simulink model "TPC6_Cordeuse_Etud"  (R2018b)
settings: Solver=ode23t  StartTime=0.0  StopTime=5  RelTol=1e-3  EnableMultiTasking=on
model workspace (MAT data in the model file):
  J = 0
  K1 = 0.561
  Kcan = 51
  Kcorde = 5052
  Ke = 0.024
  Kh = 0.0705882352941
  Ki = 0
  Kinc = 0
  Kp = 2
  Kpc = 0
  Kpot = 0.333333333333
  Kr = 0
  Kress = 0.033
  L = 0.02
  R = 0.7
  f = 0
libraries: simulink x1

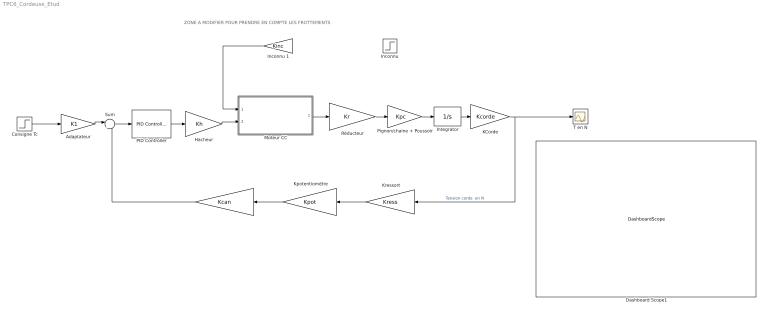
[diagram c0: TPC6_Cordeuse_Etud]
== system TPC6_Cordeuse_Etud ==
  note: ZONE A MODIFIER POUR PRENDRE EN COMPTE LES FROTTEMENTS
  " " : Gain  Gain=Kcan
  " Kpotentiomètre" : Gain  Gain=Kpot
  " Kressort" : Gain  Gain=Kress
  Adaptateur : Gain  Gain=K1
  Consigne Tc : Step  Time=0  After=250  SampleTime=0
  Dashboard Scope1 : DashboardScope  WebBlockId=46  Ymin=0  Ymax=400
  Hacheur : Gain  Gain=Kh
  "Inconnu " : Step  Time=0  After=0  SampleTime=0
  Inconnu 1 : Gain  Gain=Kinc
  Integrator : Integrator
  KCorde : Gain  Gain=Kcorde
  Moteur CC : Subsystem
  PID Controller : simulink/Continuous/PID Controller  Controller=PID  Form=Parallel  TimeDomain=Continuous-time  SampleTime=-1  IntegratorMethod=Forward Euler  FilterMethod=Forward Euler  ControllerParametersSource=internal  P=Kp  I=Ki  D=0  UseFilter=on  N=100  TunerSelectOption=Transfer Function Based (PID Tuner App)  InitialConditionSource=internal  InitialConditionForIntegrator=0  InitialConditionForFilter=0  DifferentiatorICPrevScaledInput=0  ExternalReset=none  TrackingMode=off  Kt=1  LimitOutput=off  UpperSaturationLimit=inf  LowerSaturationLimit=-inf  LinearizeAsGain=on  AntiWindupMode=none  Kb=1  POutMin=[]  POutMax=[]  IOutMin=[]  IOutMax=[]  DOutMin=[]  DOutMax=[]  NOutMin=[]  NOutMax=[]  SumOutMin=[]  SumOutMax=[]  SaturationOutMin=[]  SaturationOutMax=[]  PParamMin=[]  PParamMax=[]  IParamMin=[]  IParamMax=[]  DParamMin=[]  DParamMax=[]  NParamMin=[]  NParamMax=[]  KbParamMin=[]  KbParamMax=[]  KtParamMin=[]  KtParamMax=[]  KbOutMin=[]  KbOutMax=[]  KtOutMin=[]  KtOutMax=[]  IntegratorOutMin=[]  IntegratorOutMax=[]  FilterOutMin=[]  FilterOutMax=[]  SumI1OutMin=[]  SumI1OutMax=[]  SumI2OutMin=[]  SumI2OutMax=[]  SumI3OutMin=[]  SumI3OutMax=[]  SumI4OutMin=[]  SumI4OutMax=[]  SumDOutMin=[]  SumDOutMax=[]  DifferentiatorOutMin=[]  DifferentiatorOutMax=[]  FilterDiffOutCoefMin=[]  FilterDiffOutCoefMax=[]  ReciprocalOutMin=[]  ReciprocalOutMax=[]  SumDenOutMin=[]  SumDenOutMax=[]  SumNumOutMin=[]  SumNumOutMax=[]  DivideOutMin=[]  DivideOutMax=[]  IntegratorContinuousStateAttributes=''  IntegratorStateMustResolveToSignalObject=off  IntegratorRTWStateStorageClass=Auto  FilterContinuousStateAttributes=''  FilterStateMustResolveToSignalObject=off  FilterRTWStateStorageClass=Auto  ParallelPVariant=InternalParameters  IdealPVariant=Disabled  IVariant=InternalParameters  DVariant=InternalParameters  IntegratorVariant=Continuous  SatVariant=Disabled  AWVariant=Passthrough  PCopyVariant=Disabled  TRVariant=Disabled  FdbkBlocksVariant=Forward  IdealPFdbkVariant=Disabled  SatFdbkVariant=Disabled  DerivativeFilterVariant=ContFilter  NVariant=InternalParameters  NCopyVariant=Disabled  FilterICVariant=InternalICsFilter  IntegratorICVariant=InternalICs  ExternalResetVariant=Disabled  TRSumVariant=Passthrough  SumFdbkVariant=Disabled  SumVariant=Sum_PID
  Pignon/chaine + Poussoir : Gain  Gain=Kpc
  Réducteur : Gain  Gain=Kr
  Sum : Sum  Inputs=|+-
  T en N : Scope
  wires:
  Adaptateur/1 -> Sum/1
  Sum/1 -> PID Controller/1
  PID Controller/1 -> Hacheur/1
  Réducteur/1 -> Pignon/chaine + Poussoir/1
  Pignon/chaine + Poussoir/1 -> Integrator/1
  " "/1 -> Sum/2
  Consigne Tc/1 -> Adaptateur/1
  Integrator/1 -> KCorde/1
  " Kpotentiomètre"/1 -> " "/1
  " Kressort"/1 -> " Kpotentiomètre"/1
  ? -> Inconnu 1/1
  "Inconnu "/1 -> ?
  Inconnu 1/1 -> Moteur CC/1(In1)
  Hacheur/1 -> Moteur CC/2(In2)
  Moteur CC/1(Out1) -> Réducteur/1
  KCorde/1 -> T en N/1, " Kressort"/1  "Tension corde  en N"

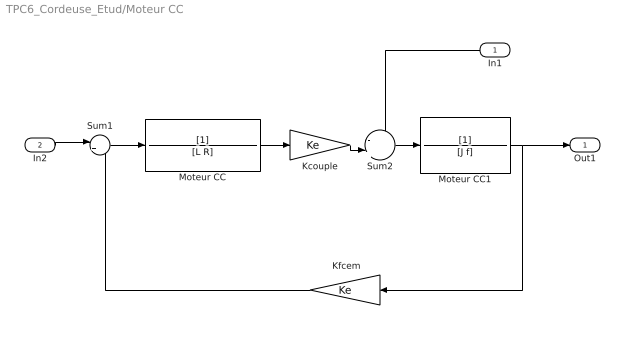
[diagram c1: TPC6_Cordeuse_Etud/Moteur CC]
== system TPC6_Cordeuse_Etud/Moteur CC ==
  In1 : Inport
  In2 : Inport  Port=2
  " Kfcem" : Gain  Gain=Ke
  Kcouple : Gain  Gain=Ke
  Moteur CC : TransferFcn  Denominator=[L R]
  Moteur CC1 : TransferFcn  Denominator=[J f]
  Sum1 : Sum  Inputs=|+-
  Sum2 : Sum  Inputs=-|+||
  Out1 : Outport
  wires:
  " Kfcem"/1 -> Sum1/2
  Moteur CC/1 -> Kcouple/1
  In2/1 -> Sum1/1
  Sum1/1 -> Moteur CC/1
  Moteur CC1/1 -> " Kfcem"/1, Out1/1
  In1/1 -> Sum2/1
  Sum2/1 -> Moteur CC1/1
  Kcouple/1 -> Sum2/2
